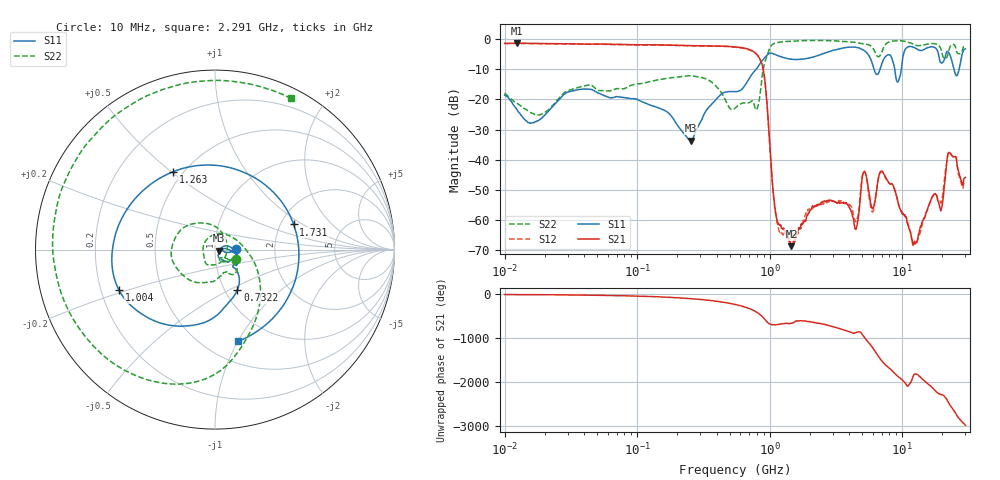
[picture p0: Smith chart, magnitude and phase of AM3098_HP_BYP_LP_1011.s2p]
!Agilent Technologies,E8364B,MY43040894,A.07.50.67
!Agilent E8364B: A.07.50.67
!Date: Wednesday, June 17, 2020 09:21:12
!Correction: S11(Full 2 Port(1,2))
!S21(Full 2 Port(1,2))
!S12(Full 2 Port(1,2))
!S22(Full 2 Port(1,2))
!S2P File: Measurements: S11, S21, S12, S22:Log Frequency Sweep
# Hz S  dB  R 50
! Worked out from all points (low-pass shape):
!   1601 points, 10 MHz to 30 GHz, reference 50 ohm
!   highest |S21| = -1.43 dB at 12.4 MHz (marker M1); lowest = -68.6 dB at 1.461 GHz (marker M2)
!   |S21| within 3 dB of the highest: start of sweep to 769.8 MHz
!   lowest |S11| = -33.6 dB at 254.7 MHz (marker M3), VSWR 1.04, Z = 52 - j0.666 ohm
!   |S11| at or under -10 dB: start of sweep to 794.3 MHz; 8.788 GHz to 9.864 GHz (1.076 GHz wide, 11.5 % of centre); 24.63 GHz to 26.91 GHz (2.285 GHz wide, 8.87 % of centre)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
!   |S22| runs from -25.2 to -0.5 dB; largest |S21 - S12| = 0.014
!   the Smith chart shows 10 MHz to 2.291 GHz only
!   S11 on the Smith chart (normalised r, x): 10 MHz: 1.27, +0.00; 732.2 MHz: 1.15, -0.55; 1.004 GHz: 0.28, -0.19; 1.263 GHz: 0.44, +0.51; 1.731 GHz: 2.35, +0.84; 2.291 GHz: 0.71, -1.00
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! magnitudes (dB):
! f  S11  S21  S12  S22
! 10 MHz  -18.6  -1.5  -1.6  -18.0
! 12.4 MHz  -23.4  -1.4  -1.5  -21.4
! 38.04 MHz  -16.7  -1.7  -1.7  -15.8
! 144.7 MHz  -22.8  -2.0  -2.0  -13.5
! 254.7 MHz  -33.6  -2.2  -2.3  -12.2
! 547.7 MHz  -17.5  -2.7  -2.8  -22.9
! 732.2 MHz  -11.8  -3.9  -4.0  -20.6
! 889.9 MHz  -6.9  -9.6  -9.7  -10.5
! 1.004 GHz  -4.7  -35.5  -35.8  -3.0
! 1.263 GHz  -6.1  -62.6  -64.8  -0.9
! 1.461 GHz  -6.7  -68.6  -64.4  -0.7
! 1.731 GHz  -6.7  -61.2  -62.2  -0.6
! 2.084 GHz  -6.1  -55.8  -56.2  -0.5
! 2.291 GHz  -5.6  -54.8  -55.3  -0.5
! 4.48 GHz  -2.8  -63.0  -60.6  -1.2
! 5.154 GHz  -3.8  -44.0  -43.8  -1.6
! 5.959 GHz  -8.2  -56.2  -57.3  -2.8
! 7.926 GHz  -5.2  -47.6  -47.7  -1.0
! 12.43 GHz  -2.9  -67.3  -67.6  -1.9
! 19.8 GHz  -8.0  -56.1  -54.0  -4.0
! 22.67 GHz  -4.8  -37.6  -37.5  -3.3
! 30 GHz  -3.3  -45.8  -47.4  -2.6
